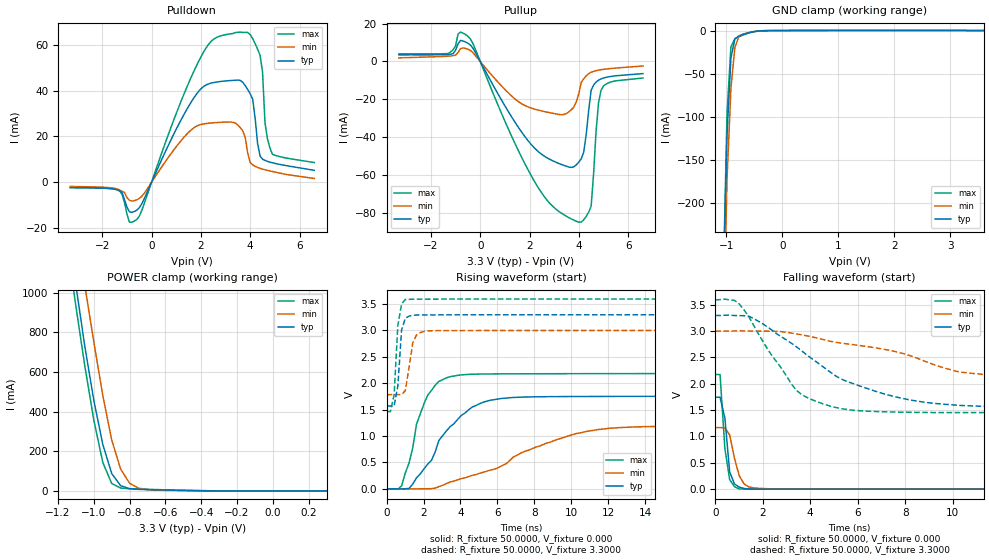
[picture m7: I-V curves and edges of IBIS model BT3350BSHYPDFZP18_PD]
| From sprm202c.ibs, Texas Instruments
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|   Model BT3350BSHYPDFZP18_PD
[Model]   BT3350BSHYPDFZP18_PD
Model_type   I/O
Polarity   Non-Inverting
Enable   Active-Low
Vinl =   1.3000V
Vinh =   1.3000V
Vmeas =   1.6500V
Cref =  15.0000pF
Rref = 100.0000M
Vref =  0.000V
C_comp   1.5700pF   1.6700pF   1.4700pF
[Model Spec]
|   typ   min   max
Vinh   1.37V   1.23V   1.59V
Vinl   1.11V   1.06V   1.23V
[Temperature Range]   25   125   -40
[Voltage Range]   3.30V   3.00V   3.60V
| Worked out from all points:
|   slope of the pulldown table from 0 to 0.495 V, typ, clamps not added: 41.7 ohm
|   slope of the pullup table from 0 to 0.495 V, typ, clamps not added: 41.6 ohm
|   GND clamp passes 1 mA (typ) near -0.48 V on its own axis
|   POWER clamp passes 1 mA (typ) near -0.38 V on its own axis
|   rising waveform, R_fixture 50.0000, V_fixture 0.000: 20-80 % time 2.13ns typ, 4.86ns min, 1.03ns max; typ from 0 V to 1.75 V
|   rising waveform, R_fixture 50.0000, V_fixture 3.3000: 20-80 % time 209ps typ, 323ps min, 221ps max; typ from 1.57 V to 3.3 V
|   falling waveform, R_fixture 50.0000, V_fixture 0.000: 20-80 % time 220ps typ, 388ps min, 255ps max; typ from 1.74 V to 0 V
|   falling waveform, R_fixture 50.0000, V_fixture 3.3000: 20-80 % time 3.86ns typ, 8.73ns min, 1.86ns max; typ from 3.3 V to 1.55 V
[Pulldown]
| voltage   I(typ)   I(min)   I(max)
-3.3V     -2.395mA   -1.898mA   -2.403mA
-1.3V     -3.811mA   -3.398mA   -3.788mA
-900mV    -12.97mA   -7.916mA   -17.55mA
-600mV    -12.26mA   -7.745mA   -16.35mA
2V        40.86mA    25.24mA    54.83mA
3.5V      44.7mA     24.98mA    65.62mA
4.1V      36.36mA    7.585mA    62.88mA
4.4V      11.43mA    6.058mA    55.64mA
4.5V      10.06mA    5.732mA    48.29mA
4.6V      9.513mA    5.439mA    26.03mA
4.9V      8.477mA    4.664mA    12.22mA
6.6V      5.171mA    1.589mA    8.568mA
[Pullup]
| voltage   I(typ)   I(min)   I(max)
-3.3V     3.472mA    1.905mA    4.03mA
-1.3V     3.654mA    2.79mA     4.197mA
-900mV    9.239mA    4.707mA    14.45mA
-500mV    9.64mA     6.478mA    13.31mA
1.9V      -41.21mA   -23.8mA    -56.28mA
3.4V      -54.97mA   -28.03mA   -81.11mA
4V        -53.19mA   -17mA      -84.98mA
4.2V      -47.87mA   -9.18mA    -83.7mA
4.5V      -15.17mA   -5.708mA   -76.52mA
4.7V      -10.89mA   -4.857mA   -36.83mA
4.9V      -9.244mA   -4.36mA    -15.23mA
6.6V      -6.422mA   -2.393mA   -8.758mA
[GND_clamp]
| voltage   I(typ)   I(min)   I(max)
-3.3V     -17.96A    -16.59A    -18.96A
-1.06V    -298.5mA   -373.9mA   -299.9mA
-990mV    -120.1mA   -172.1mA   -95.79mA
-920mV    -31.73mA   -66.52mA   -18.62mA
-850mV    -9.689mA   -19.82mA   -9.524mA
-780mV    -6.264mA   -7.057mA   -7.298mA
-710mV    -4.678mA   -4.122mA   -5.409mA
-640mV    -3.321mA   -2.906mA   -3.657mA
-500mV    -1.166mA   -1.265mA   -996.7uA
-360mV    -227.4uA   -292.7uA   -191.5uA
3.6V      0A         0A         0A
[POWER_clamp]
| voltage   I(typ)   I(min)   I(max)
-3.3V     16.8A      15.72A     17.64A
-1.15V    1.371A     1.626A     1.251A
-1.1V     1.036A     1.326A     930.3mA
-1.05V    727.5mA    1.034A     628.8mA
-1V       456.7mA    751.3mA    357.1mA
-950mV    235.2mA    481.7mA    144.1mA
-900mV    87.65mA    256.7mA    37.39mA
-850mV    26.21mA    109.7mA    14.54mA
-800mV    11.29mA    38.62mA    10.91mA
-750mV    7.906mA    13.87mA    9.375mA
-650mV    5.494mA    4.052mA    6.775mA
300mV     0A         0A         0A
[Ramp]
| variable   typ   min   max
dV/dt_r   1.0511/2.1345n   0.7104/4.8688n   1.3095/1.0535n
dV/dt_f   1.0462/3.8249n   0.6032/6.1173n   1.2841/1.8435n
R_load = 50.0000
[Rising Waveform]
R_fixture = 50.0000
V_fixture = 0.000
V_fixture_min = 0.000
V_fixture_max = 0.000
| time   V(typ)   V(min)   V(max)
0s        8.349uV    2.65uV     13.55uV
808.1ps   -4.907mV   -72.55uV   54.95mV
1.414ns   88.49mV    -3.42mV    776.3mV
1.616ns   206.8mV    -2.07mV    1.22V
2.222ns   465.6mV    557.2uV    1.772V
3.434ns   1.175V     126.7mV    2.124V
4.646ns   1.55V      255.3mV    2.171V
5.657ns   1.681V     357.2mV    2.176V
10.91ns   1.749V     1.092V     2.181V
20ns      1.752V     1.183V     2.183V
[Rising Waveform]
R_fixture = 50.0000
V_fixture = 3.3000
V_fixture_min = 3.0000
V_fixture_max = 3.6000
| time   V(typ)   V(min)   V(max)
0s        1.569V     1.783V     1.462V
202ps     1.569V     1.783V     1.462V
404ps     1.571V     1.784V     1.777V
606.1ps   1.946V     1.784V     3.097V
808.1ps   3.006V     1.784V     3.5V
1.01ns    3.229V     1.859V     3.587V
1.414ns   3.289V     2.764V     3.591V
1.616ns   3.292V     2.915V     3.592V
2.02ns    3.294V     2.982V     3.593V
20ns      3.297V     2.999V     3.595V
[Falling Waveform]
R_fixture = 50.0000
V_fixture = 0.000
V_fixture_min = 0.000
V_fixture_max = 0.000
| time   V(typ)   V(min)   V(max)
0s        1.744V     1.169V     2.177V
202ps     1.745V     1.169V     2.175V
404ps     1.352V     1.163V     773.3mV
606.1ps   327.3mV    1.03V      182.2mV
808.1ps   99.12mV    587.2mV    48.01mV
1.01ns    38.64mV    254.1mV    4.085mV
1.212ns   13.22mV    100.9mV    916.2uV
1.414ns   3.098mV    42.99mV    742.1uV
2.424ns   440.4uV    5.011mV    183.2uV
20ns      -1.523uV   12.18uV    -1.525uV
[Falling Waveform]
R_fixture = 50.0000
V_fixture = 3.3000
V_fixture_min = 3.0000
V_fixture_max = 3.6000
| time   V(typ)   V(min)   V(max)
0s        3.297V     2.999V     3.595V
808.1ps   3.295V     3.002V     3.584V
1.01ns    3.293V     3.006V     3.514V
1.616ns   3.239V     2.999V     3.11V
3.434ns   2.696V     2.945V     1.869V
5.051ns   2.156V     2.789V     1.553V
7.273ns   1.789V     2.641V     1.467V
9.495ns   1.617V     2.322V     1.454V
10.51ns   1.585V     2.213V     1.454V
20ns      1.553V     1.788V     1.456V
